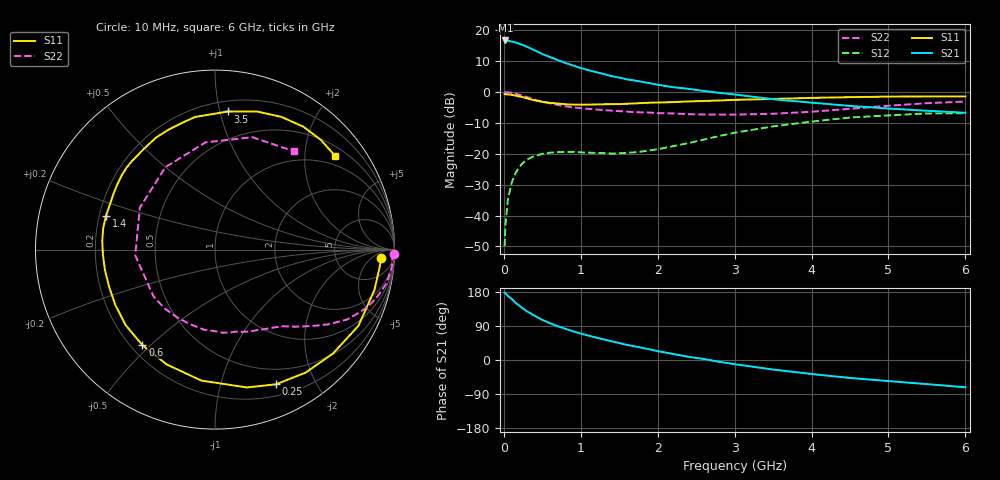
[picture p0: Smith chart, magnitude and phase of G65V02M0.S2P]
! SIEMENS Small Signal Semiconductors
! BFG193
! Si NPN RF Bipolar Junction Transistor in SOT223
! VCE = 5 V  IC = 2 mA
! Common Emitter S-Parameters:  August  1996
# GHz  S  MA  R  50
!  f  S11  S21  S12  S22
! GHz  MAG  ANG  MAG  ANG  MAG  ANG  MAG  ANG
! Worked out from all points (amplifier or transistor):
!   36 points, 10 MHz to 6 GHz, reference 50 ohm
!   highest |S21| = 16.7 dB at 20 MHz (marker M1)
!   |S21| within 3 dB of that: start of sweep to 384.4 MHz
!   unconditionally stable (mu >= 1): 1.371 GHz to 2.542 GHz
!   at 250 MHz: K = 0.17, MSG = 19.0 dB, |S12| = -22.9 dB
!   at 1.4 GHz: K = 1.03, MAG = 11.5 dB, |S12| = -19.9 dB
!   at 6 GHz: K = 0.95, MSG = 0.1 dB, |S12| = -6.9 dB
!   S11 on the Smith chart (normalised r, x): 10 MHz: 19, -12; 250 MHz: 0.32, -1.50; 600 MHz: 0.25, -0.47; 1.4 GHz: 0.23, +0.14; 3.5 GHz: 0.28, +1.06; 6 GHz: 0.73, +2.73
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0.01  0.9284 -2.8  6.745 177.8  0.0032 92.9  0.9969 -1.3
0.02  0.9226 -5.9  6.84 176.8  0.0067 88.6  0.9893 -2.2
0.05  0.9165 -14.2  6.782 169.6  0.0173 81.7  0.9901 -5.7
0.1  0.9049 -28.0  6.592 161.6  0.0335 75.9  0.9735 -11.2
0.15  0.876 -41.4  6.352 151.4  0.0483 66.8  0.941 -16.3
0.25  0.8238 -65.7  5.743 135.7  0.0717 54.5  0.8659 -24.6
0.3  0.7882 -77.0  5.409 128.6  0.0804 49.6  0.8312 -28.0
0.4  0.7338 -95.9  4.744 116.9  0.0924 40.6  0.7564 -33.4
0.5  0.6942 -112.8  4.122 105.8  0.0998 33.7  0.699 -37.4
0.6  0.6682 -127.3  3.685 97.2  0.1044 29.0  0.6556 -40.7
0.7  0.6519 -139.7  3.304 89.3  0.1064 25.2  0.62 -43.9
0.8  0.6354 -151.0  2.955 82.2  0.1074 22.4  0.5889 -46.6
0.9  0.6254 -160.5  2.683 75.7  0.1075 20.4  0.5657 -49.0
1.1  0.6249 -177.2  2.256 64.4  0.1046 18.7  0.5337 -55.1
1.4  0.636 162.7  1.807 49.4  0.1014 20.3  0.5008 -64.7
1.6  0.6454 151.2  1.605 39.9  0.1037 24.2  0.4824 -72.1
2.2  0.6873 125.1  1.2 15.9  0.1327 34.1  0.4501 -98.0
2.8  0.7301 104.4  0.972 -4.7  0.1941 32.5  0.4316 -130.8
3.5  0.773 84.6  0.765 -25.1  0.278 18.4  0.4455 -175.9
4.5  0.8269 63.4  0.596 -47.4  0.3869 -6.1  0.5357 121.1
5.5  0.8493 46.1  0.498 -63.6  0.4511 -35.4  0.6601 71.6
6  0.8491 38.0  0.462 -72.0  0.4537 -51.0  0.7022 51.3
